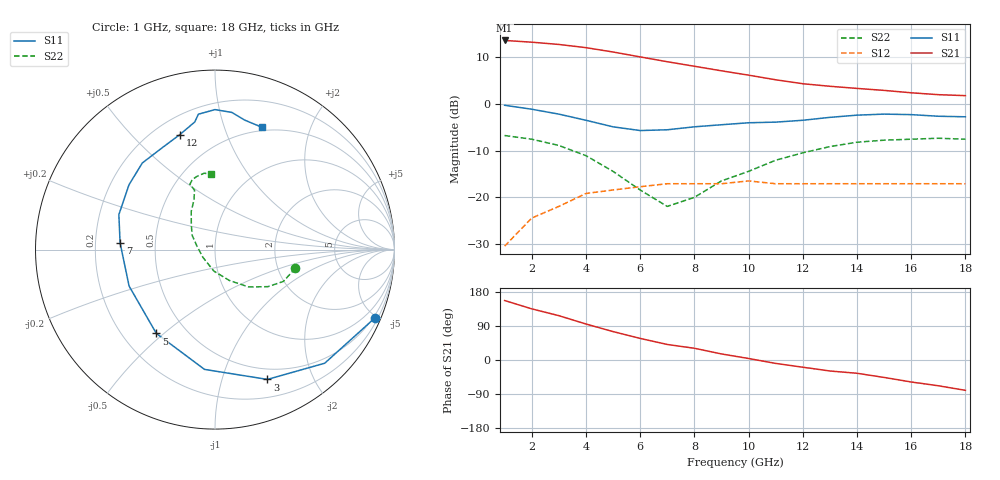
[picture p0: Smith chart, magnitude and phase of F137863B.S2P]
!ATF-13786
!S-PARAMETERS at Vds=3V  Id=40mA.  LAST UPDATED 07-22-92
# ghz s ma r 50
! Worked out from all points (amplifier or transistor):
!   18 points, 1 GHz to 18 GHz, reference 50 ohm
!   highest |S21| = 13.6 dB at 1 GHz (marker M1)
!   |S21| within 3 dB of that: start of sweep to 5.502 GHz
!   unconditionally stable (mu >= 1): 5.845 GHz to 14.94 GHz; 15.15 GHz to end of sweep
!   at 4 GHz: K = 0.75, MSG = 15.6 dB, |S12| = -19.2 dB
!   at 10 GHz: K = 1.14, MAG = 9.1 dB, |S12| = -16.5 dB
!   at 18 GHz: K = 1.16, MAG = 7.0 dB, |S12| = -17.1 dB
!   S11 on the Smith chart (normalised r, x): 1 GHz: 0.38, -4.89; 3 GHz: 0.38, -1.41; 5 GHz: 0.34, -0.47; 7 GHz: 0.31, +0.03; 12 GHz: 0.30, +0.70; 18 GHz: 0.46, +1.35
1  0.97 -23.0  4.8 157.0  0.03 77.0  0.46 -13.0
2  0.88 -46.0  4.6 135.0  0.06 66.0  0.42 -25.0
3  0.78 -68.0  4.35 117.0  0.08 58.0  0.36 -35.0
4  0.67 -95.0  4.02 95.0  0.11 47.0  0.28 -48.0
5  0.57 -125.0  3.61 75.0  0.12 37.0  0.19 -65.0
6  0.52 -157.0  3.2 57.0  0.13 28.0  0.12 -93.0
7  0.53 176.0  2.84 41.0  0.14 21.0  0.08 -147.0
8  0.57 160.0  2.54 31.0  0.14 18.0  0.1 171.0
9  0.6 143.0  2.27 16.0  0.14 12.0  0.15 148.0
10  0.63 130.0  2.04 4.0  0.15 6.0  0.19 134.0
11  0.64 117.0  1.82 -9.0  0.14 0.0  0.25 122.0
12  0.67 107.0  1.65 -19.0  0.14 -4.0  0.3 113.0
13  0.72 99.0  1.55 -29.0  0.14 -8.0  0.35 109.0
14  0.76 97.0  1.47 -35.0  0.14 -9.0  0.39 111.0
15  0.78 90.0  1.4 -46.0  0.14 -14.0  0.41 108.0
16  0.77 83.0  1.32 -58.0  0.14 -20.0  0.42 104.0
17  0.74 77.0  1.26 -68.0  0.14 -28.0  0.43 98.0
18  0.73 69.0  1.23 -80.0  0.14 -36.0  0.42 93.0
